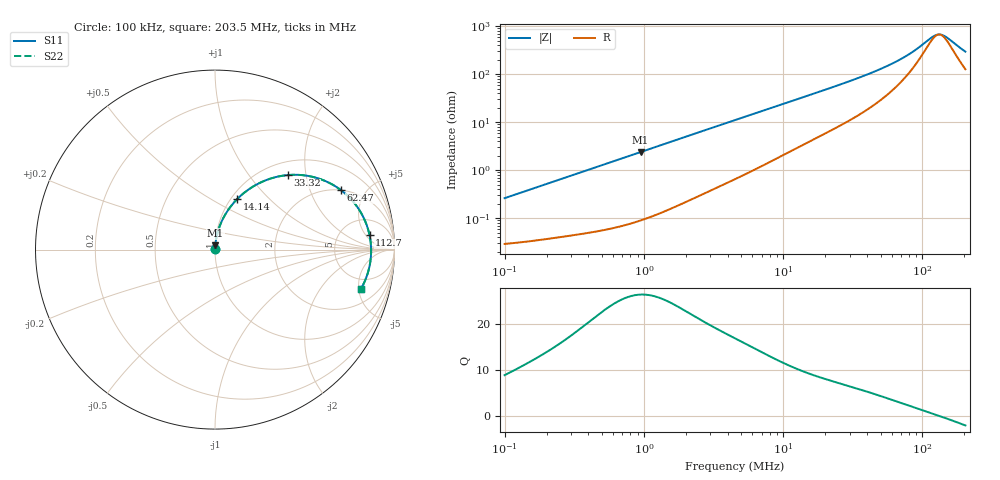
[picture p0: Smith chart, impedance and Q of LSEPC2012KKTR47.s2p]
! LSEPC2012KKTR47  S-PARAMETER MODEL  ( General Type )
! Model Generated by TAIYO YUDEN Corporation (http://www.ty-top.com)
! Version 1.0
! TAIYO YUDEN Control No. 180907NI43SB-FBB
! Copyright(c) 2018 TAIYO YUDEN CO.,LTD. All Rights Reserved.
! Product Description (link to TY-COMPAS)
! https://ds.yuden.co.jp/TYCOMPAS/or/detail?pn=LSEPC2012KKTR47M&u=M
! Products Name : Inductors
! Characteristics :
!  Inductance : 0.47 uH , SRF(min) : -Hz , DC Resistance(max) : 0.03 Ohm
!  Rated Current : Saturation :4500 mA , Temp Rise : 4200 mA (40 degC)
!  Case Size : 2.0 x 1.2 / 0.079 x 0.047 [mm/inch] , Thickness : 1 / 0.039 [mm/inch]
!  (Conditions: Temperature = 25 degC , DC Bias Current/Voltage = 0A / 0V)
! External Node Assignments :
!  1  o---GGG---o  2
! GND o---------o GND
! Frequency Range : 0.1MHz  -  203.457813MHz  [ 402 STEP ]
# MHz S RI R 50
! Freq[MHz].  S11 Real  S11 Imag  S21 Real  S21 Imag  S12 Real  S12 Imag  S22 Real  S22 Imag
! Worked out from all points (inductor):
!   401 points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, 100 kHz to 203.5 MHz, reference 50 ohm
!   read as one part in series: L = 414 nH near 103.9 kHz
!   highest Q = 26.5 at 946.2 kHz (marker M1), where L = 401 nH
!   self-resonance near 131.7 MHz
!   S11 on the Smith chart (normalised r, x): 100 kHz: 1.00, +0.01; 14.14 MHz: 1.07, +0.67; 33.32 MHz: 1.26, +1.58; 62.47 MHz: 1.99, +3.31; 112.7 MHz: 10, +6; 203.5 MHz: 3.53, -5.30
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0.1  0.0003 0.00261  0.9997 -0.00261  0.9997 -0.00261  0.0003 0.00261
0.358236  0.000556 0.00913  0.9994 -0.00913  0.9994 -0.00913  0.000556 0.00913
0.946237  0.00147 0.0238  0.9985 -0.0238  0.9985 -0.0238  0.00147 0.0238
1.283332  0.00228 0.0321  0.9977 -0.0321  0.9977 -0.0321  0.00228 0.0321
2.547426  0.00694 0.0626  0.9931 -0.0626  0.9931 -0.0626  0.00694 0.0626
4.51063  0.0183 0.1076  0.9817 -0.1076  0.9817 -0.1076  0.0183 0.1076
8.619012  0.0554 0.1924  0.9446 -0.1924  0.9446 -0.1924  0.0554 0.1924
14.14192  0.1249 0.2828  0.8751 -0.2828  0.8751 -0.2828  0.1249 0.2828
16.15871  0.1534 0.309  0.8466 -0.309  0.8466 -0.309  0.1534 0.309
23.2038  0.2578 0.3756  0.7422 -0.3756  0.7422 -0.3756  0.2578 0.3756
33.32052  0.4044 0.4151  0.5956 -0.4151  0.5956 -0.4151  0.4044 0.4151
44.33835  0.5408 0.4061  0.4592 -0.4061  0.4592 -0.4061  0.5408 0.4061
57.88634  0.6667 0.3551  0.3333 -0.3551  0.3333 -0.3551  0.6667 0.3551
62.46847  0.6996 0.333  0.3004 -0.333  0.3004 -0.333  0.6996 0.333
83.12442  0.8014 0.2249  0.1986 -0.2249  0.1986 -0.2249  0.8014 0.2249
94.97886  0.8343 0.164  0.1657 -0.164  0.1657 -0.164  0.8343 0.164
112.7373  0.8612 0.0796  0.1388 -0.0796  0.1388 -0.0796  0.8612 0.0796
126.3848  0.869 0.0211  0.131 -0.0211  0.131 -0.0211  0.869 0.0211
139.0115  0.8693 -0.0281  0.1307 0.0281  0.1307 0.0281  0.8693 -0.0281
150.0152  0.8654 -0.0675  0.1346 0.0675  0.1346 0.0675  0.8654 -0.0675
188.534  0.8319 -0.1821  0.1681 0.1821  0.1681 0.1821  0.8319 -0.1821
203.4578  0.8135 -0.2181  0.1865 0.2181  0.1865 0.2181  0.8135 -0.2181
